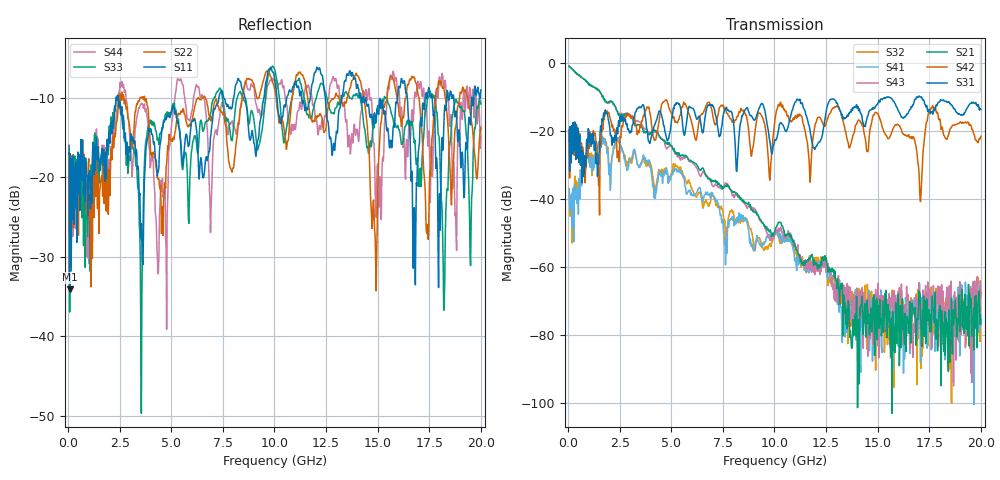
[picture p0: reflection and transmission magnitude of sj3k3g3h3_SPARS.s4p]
! FILE: E:\users\goganessyan\GBX_Backplane\FR408_backplane\1m_OUTBOUND_TRU\sj3k3g3h3_SPARS.s4p
# MHZ S RI R 50.00
! FREQ  S11  S12  S13  S14
!  S21  S22  S23  S24
!  S31  S32  S33  S34
!  S41  S42  S43  S44
!  REAL  IMAG  REAL  IMAG  REAL  IMAG  REAL  IMAG
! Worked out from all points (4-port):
!   799 points, 50 MHz to 20 GHz, reference 50 ohm
!   strongest paths, dB at 50 MHz, 5.025 GHz, 10.03 GHz, 15.03 GHz, 20 GHz:
!     S31: -19.7, -16.3, -22.6, -11.9, -13.8
!     S42: -19.9, -15.2, -16.7, -15.2, -21.7
!     S21: -1.0, -24.4, -49.2, -71.4, -76.9
!     S43: -1.1, -24.8, -50.5, -64.8, -68.8
!     S41: -37.0, -32.7, -50.2, -83.3, -75.4
!     S32: -37.6, -31.8, -50.6, -78.4, -66.7
!   lowest |S11| = -34.1 dB at 75 MHz (marker M1), VSWR 1.04, Z = 52 + j0.0948 ohm
!   |S11| at or under -10 dB: start of sweep to 2.324 GHz; 2.441 GHz to 7.308 GHz (4.868 GHz wide, 99.9 % of centre); 14.43 GHz to 15.96 GHz (1.537 GHz wide, 10.1 % of centre)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
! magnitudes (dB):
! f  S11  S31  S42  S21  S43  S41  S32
! 50 MHz  -16.1  -19.7  -19.9  -1.0  -1.1  -37.0  -37.6
! 75 MHz  -34.1  -31.8  -33.9  -1.1  -1.1  -41.9  -41.1
! 2.425 GHz  -9.7  -18.6  -26.0  -15.2  -14.9  -22.1  -22.5
! 3.55 GHz  -25.8  -13.1  -17.9  -19.0  -18.0  -29.8  -29.5
! 13.53 GHz  -6.9  -15.4  -22.6  -78.2  -64.9  -68.8  -68.8
! 18.23 GHz  -12.0  -11.3  -21.6  -80.0  -74.4  -74.5  -72.2
! 20 GHz  -9.0  -13.8  -21.7  -76.9  -68.8  -75.4  -66.7
